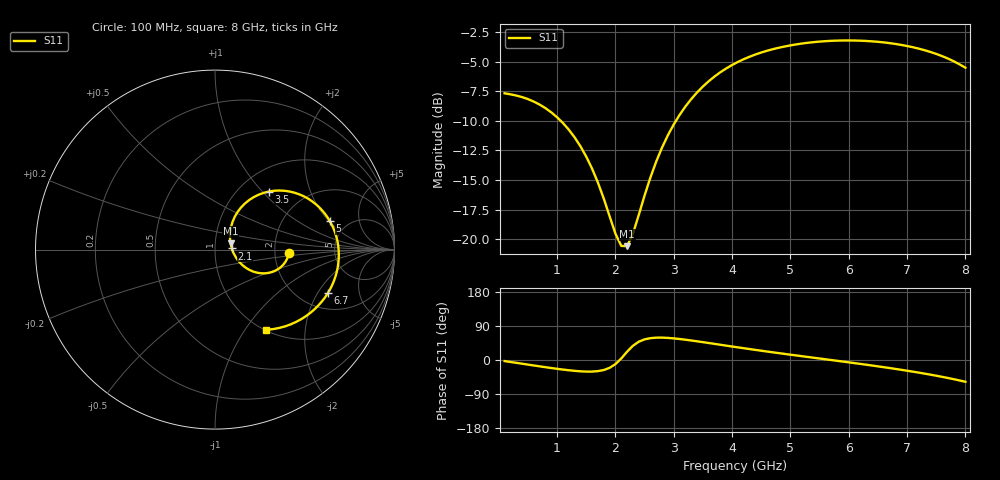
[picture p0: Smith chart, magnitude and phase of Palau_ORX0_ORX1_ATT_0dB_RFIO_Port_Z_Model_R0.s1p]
! Created Fri Jul 10 10:22:44 2020
! Palau ORX0/ORX1 RFIO Port Impedance Model.
! Attenuation : 0 dB.
! Revision		: R0.
! Impedance Mode 	: Balanced Differential-Mode.
! Impedance Format 	: Series Equivalent Differential Impedance (SEDZ).
# hz S ma R 50
! 1 Port Network Data from SP1.SP block
! freq  magS11  angS11
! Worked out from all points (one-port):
!   80 points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, 100 MHz to 8 GHz, reference 50 ohm
!   lowest |S11| = -20.6 dB at 2.2 GHz (marker M1), VSWR 1.21, Z = 59.3 + j4.18 ohm
!   |S11| at or under -10 dB: 1.062 GHz to 3.037 GHz (1.975 GHz wide, 96.4 % of centre)
!   S11 on the Smith chart (normalised r, x): 100 MHz: 2.40, -0.12; 2.1 GHz: 1.21, +0.02; 3.5 GHz: 1.36, +1.09; 5 GHz: 3.64, +2.05; 6.7 GHz: 2.76, -2.47; 8 GHz: 1.01, -1.26
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1e8  0.4136 -2.9
6e8  0.3815 -14.4
9e8  0.3435 -21.2
1.1e9  0.3096 -25.3
1.4e9  0.2469 -29.8
1.6e9  0.1985 -30.5
1.8e9  0.1484 -26.4
2e9  0.1055 -10.9
2.1e9  0.09367 4.1
2.2e9  0.09342 21.9
2.3e9  0.1055 37.6
2.5e9  0.1531 54.4
2.7e9  0.213 59.0
2.9e9  0.275 58.3
3.1e9  0.335 55.4
3.5e9  0.4418 47.1
3.8e9  0.5076 40.2
4.1e9  0.561 33.3
4.6e9  0.6255 22.3
5e9  0.6589 14.0
5.1e9  0.6654 12.0
5.6e9  0.6866 1.9
6.1e9  0.6909 -8.3
6.4e9  0.6854 -14.6
6.7e9  0.6738 -21.2
7.1e9  0.6472 -30.7
7.6e9  0.5937 -44.4
8e9  0.5305 -57.5
